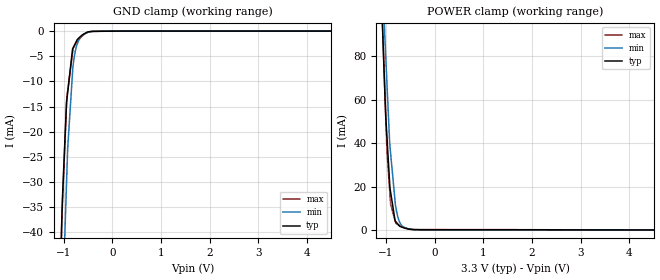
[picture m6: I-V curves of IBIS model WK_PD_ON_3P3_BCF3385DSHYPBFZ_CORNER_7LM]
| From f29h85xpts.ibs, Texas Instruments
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|   Model Cell WK_PD_ON_3P3_BCF3385DSHYPBFZ_CORNER_7LM
|WK_PD_ON_3P3_BCF3385DSHYPBFZ_CORNER_7LM
[Model]   WK_PD_ON_3P3_BCF3385DSHYPBFZ_CORNER_7LM
Model_type   Input
Polarity   Non-Inverting
Vinl = 0.8
Vinh = 2
|   typ   min   max
C_comp   0.44pF   0.4pF   0.46pF
[Model Spec]
Vinl   0.8   0.8   0.8
Vinh   2   2   2
[Temperature Range]   25   155   -40
[Voltage Range]   3.3   2.8   3.63
| Nom Voltages:
|   VDD=1.23, VDDS=3.3, VSS=0
| Min Voltages:
|   VDD=1.08, VDDS=2.8, VSS=0
| Max Voltages:
|   VDD=1.32, VDDS=3.63, VSS=0
[Power Clamp Reference]   3.3   2.8   3.63
[GND Clamp Reference]   0   0   0
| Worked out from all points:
|   GND clamp passes 1 mA (typ) near -0.64 V on its own axis
|   POWER clamp passes 1 mA (typ) near -0.64 V on its own axis
[GND Clamp]
|   Voltage   I(typ)   I(min)   I(max)
-3.3V     -1.475A    -1.211A    -2.162A
-1.048V   -42.94mA   -65.58mA   -41.41mA
-1.04V    -39.5mA    -62.39mA   -38.41mA
-1.014V   -31.27mA   -52.41mA   -32.3mA
-939.6mV  -14.29mA   -30.41mA   -14.69mA
-932.9mV  -13.72mA   -28.44mA   -13.12mA
-915.9mV  -12.25mA   -23.41mA   -11.86mA
-809.2mV  -3.443mA   -7.259mA   -3.972mA
-759.5mV  -2.476mA   -4mA       -2.689mA
-688.5mV  -1.384mA   -1.803mA   -1.754mA
-516.9mV  -223.8uA   -295.8uA   -313.6uA
6.6V      0A         0A         0A
[POWER Clamp]
|   Voltage   I(typ)   I(min)   I(max)
-3.3V     1.946A     2.25A      2.109A
-1.078V   96.56mA    126.6mA    98.47mA
-1.036V   70.43mA    96.04mA    71.34mA
-1.025V   63.27mA    88.85mA    63.91mA
-1.004V   51.2mA     78.46mA    50.3mA
-979.5mV  41.84mA    66.39mA    35.68mA
-926.1mV  21.42mA    40.05mA    18.2mA
-906.9mV  17.45mA    35.42mA    11.92mA
-809.2mV  4.076mA    11.8mA     3.754mA
-685.9mV  1.378mA    2.25mA     1.667mA
-260.1mV  131uA      51.42uA    166uA
6.6V      0A         0A         0A
